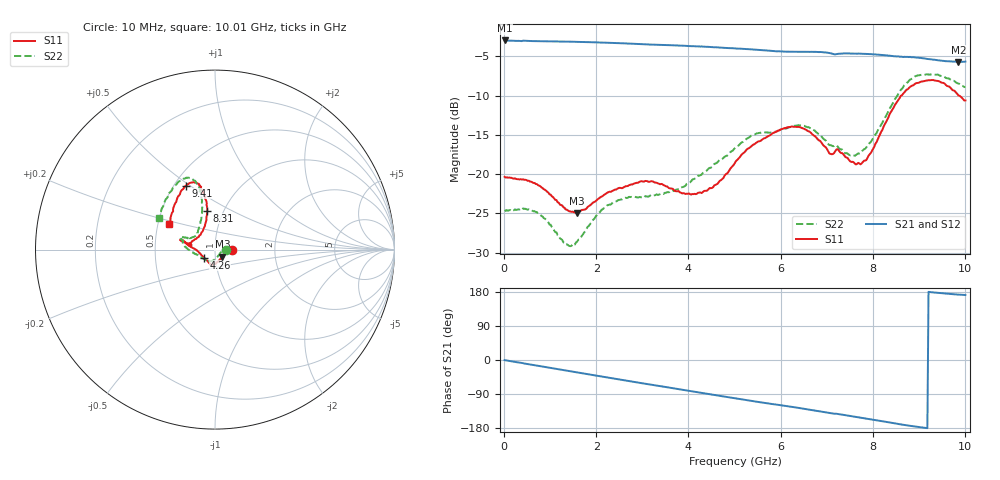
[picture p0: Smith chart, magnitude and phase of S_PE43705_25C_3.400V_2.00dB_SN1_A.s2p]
! Device ID: PE43705
! Serial: 1
! Insertion: A
! Impedance: 50 ohm
! Temp: 25C
! VDD: 3.400V
! Attenuation Step: 2.00dB
#  Hz  S  RI  R  50
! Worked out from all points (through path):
!   401 points, 10 MHz to 10.01 GHz, reference 50 ohm
!   highest |S21| = -2.99 dB at 10 MHz (marker M1); lowest = -5.7 dB at 9.86 GHz (marker M2)
!   group delay of S21, straight-line fit = 53.6 ps
!   lowest |S11| = -24.9 dB at 1.585 GHz (marker M3), VSWR 1.12, Z = 54.1 - j4.26 ohm
!   |S11| at or under -10 dB: start of sweep to 8.619 GHz; 9.86 GHz to end of sweep
!   |S22| runs from -29.2 to -7.3 dB; largest |S21 - S12| = 0.0059
!   S11 on the Smith chart (normalised r, x): 10 MHz: 1.21, -0.00; 4.26 GHz: 0.88, -0.08; 8.31 GHz: 0.84, +0.38; 9.41 GHz: 0.57, +0.48; 10.01 GHz: 0.57, +0.18
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1e7  0.096 -0.000614  0.7084 -0.00363  0.7088 -0.00314  0.0591 -0.000282
6.6e8  0.0872 0.01  0.682 -0.1667  0.6819 -0.1664  0.056 0.0152
1.335e9  0.0556 -0.0213  0.6174 -0.3226  0.6175 -0.3222  0.033 -0.0133
1.585e9  0.0408 -0.0393  0.5835 -0.3753  0.5838 -0.3752  0.022 -0.0301
1.685e9  0.0354 -0.0474  0.5692 -0.3953  0.5692 -0.3953  0.0158 -0.0372
2.31e9  0.00442 -0.0769  0.462 -0.5045  0.4621 -0.5041  -0.0141 -0.0624
3.36e9  -0.0252 -0.0831  0.2439 -0.618  0.2447 -0.6174  -0.0423 -0.0607
4.26e9  -0.062 -0.0446  0.0427 -0.6469  0.0429 -0.6462  -0.0924 -0.0338
5.01e9  -0.1177 0.00672  -0.1202 -0.619  -0.1195 -0.6193  -0.1464 -0.000754
5.435e9  -0.1526 0.0273  -0.2038 -0.5858  -0.2034 -0.5865  -0.176 0.0294
6.035e9  -0.1855 0.0552  -0.3005 -0.5226  -0.2982 -0.5231  -0.1862 0.0549
6.685e9  -0.1746 0.0413  -0.4024 -0.444  -0.4026 -0.4437  -0.1788 0.0704
7.085e9  -0.1315 0.0272  -0.4534 -0.374  -0.4539 -0.3747  -0.1421 0.0564
7.26e9  -0.1366 0.037  -0.4636 -0.3535  -0.4621 -0.3543  -0.1312 0.0658
7.685e9  -0.0881 0.0783  -0.5122 -0.2822  -0.5113 -0.2824  -0.0995 0.0916
7.91e9  -0.0647 0.1139  -0.5288 -0.2382  -0.5288 -0.2414  -0.0887 0.1268
8.31e9  -0.0438 0.2173  -0.5462 -0.1601  -0.5442 -0.163  -0.0716 0.2307
8.36e9  -0.0437 0.2343  -0.5472 -0.1492  -0.5457 -0.1515  -0.0722 0.2494
8.86e9  -0.0876 0.3554  -0.5517 -0.0527  -0.5491 -0.056  -0.1221 0.3885
9.41e9  -0.1611 0.3567  -0.5297 0.0272  -0.5284 0.0267  -0.2029 0.379
9.86e9  -0.2332 0.2135  -0.5129 0.0666  -0.5128 0.0661  -0.2887 0.2414
1.001e10  -0.2558 0.145  -0.5143 0.077  -0.5154 0.0758  -0.3131 0.1742
